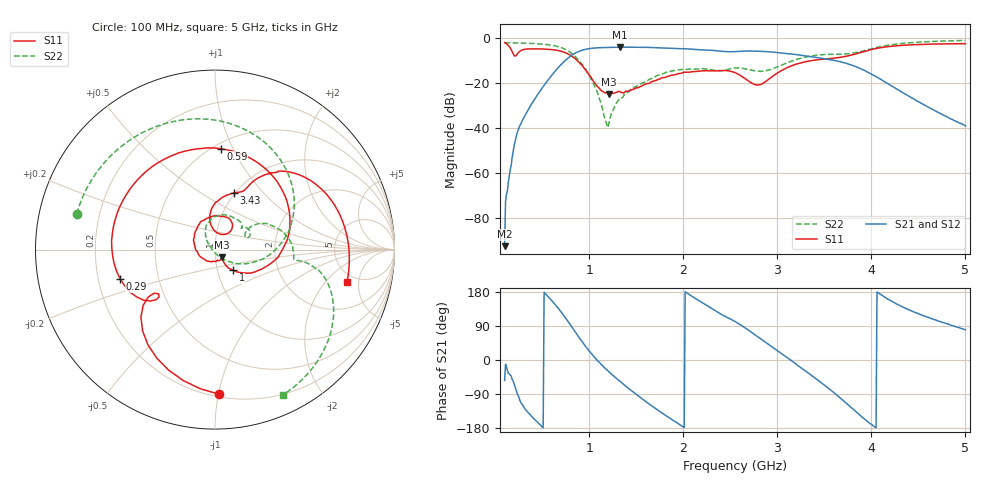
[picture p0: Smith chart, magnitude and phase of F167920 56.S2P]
!  2-Port S-parameters saved by WinCal
! VAR MeasName=S-Parameters (CALIBRATED_DATA) read from VNA (N5242A)
! VAR MeasDate=2016-11-22 9:58:16
! VAR NAME=F167920 56
! VAR FILENAME=F167920 56.S2P
! VAR DATE=2016-11-22 9:58:16
! VAR PHYS_PORTS=1,2
# Hz S DB R 50
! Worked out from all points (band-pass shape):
!   491 points, 100 MHz to 5 GHz, reference 50 ohm
!   highest |S21| = -3.95 dB at 1.33 GHz (marker M1); lowest = -92.6 dB at 100 MHz (marker M2)
!   |S21| within 3 dB of the highest: 838.6 MHz to 3.138 GHz (2.299 GHz wide, 116 % of centre)
!   lowest |S11| = -24.7 dB at 1.21 GHz (marker M3), VSWR 1.12, Z = 53.7 - j4.7 ohm
!   |S11| at or under -10 dB: 873.3 MHz to 3.356 GHz (2.483 GHz wide, 117 % of centre)
!   |S22| runs from -39.7 to -1.0 dB; largest |S21 - S12| = 0.001
!   S11 on the Smith chart (normalised r, x): 100 MHz: 0.22, -1.01; 290 MHz: 0.29, -0.14; 590 MHz: 0.54, +0.90; 1 GHz: 1.19, -0.28; 3.43 GHz: 0.99, +0.70; 5 GHz: 4.20, -3.51
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1e8  -1.86 -88.2  -92.59 -53.9  -80.56 1.6  -1.98 165.5
1.5e8  -3.76 -125.2  -61.21 -36.2  -61.52 -49.6  -2.01 158.2
2e8  -7.59 -144.4  -48.13 -62.1  -48.26 -63.1  -2.05 150.8
2.9e8  -5.14 -162.8  -36.46 -118.8  -36.55 -119.0  -2.15 137.0
4.1e8  -4.71 148.4  -27.74 -154.5  -27.73 -154.7  -2.36 117.3
5.9e8  -4.98 86.8  -17.07 160.0  -17.06 160.0  -3.05 81.9
7.5e8  -6.51 30.1  -9.71 110.3  -9.70 110.3  -5.05 40.0
9.2e8  -11.88 -29.3  -5.37 50.0  -5.36 50.0  -11.43 -11.6
1e9  -16.37 -48.9  -4.62 23.7  -4.62 23.7  -16.51 -31.9
1.18e9  -24.31 -47.7  -4.10 -24.4  -4.10 -24.4  -37.56 -120.5
1.21e9  -24.75 -48.9  -4.07 -31.5  -4.06 -31.5  -37.79 -172.5
1.33e9  -23.96 -72.6  -3.95 -57.3  -3.95 -57.3  -27.26 135.6
1.74e9  -18.24 161.5  -4.25 -134.0  -4.25 -134.0  -16.35 105.8
2.07e9  -15.10 107.9  -4.83 171.8  -4.83 171.8  -13.72 63.4
2.55e9  -15.27 55.6  -5.92 101.7  -5.93 101.6  -13.24 31.5
2.8e9  -20.75 75.7  -5.77 60.1  -5.77 60.1  -14.66 22.0
3.08e9  -13.59 97.0  -6.67 10.6  -6.68 10.6  -11.35 31.5
3.37e9  -9.89 75.3  -8.27 -41.8  -8.27 -41.8  -7.80 10.9
3.43e9  -9.55 71.4  -8.64 -52.8  -8.65 -52.8  -7.48 6.1
3.81e9  -7.23 60.7  -12.23 -130.8  -12.23 -130.8  -6.59 -7.5
4.19e9  -3.66 36.0  -20.58 158.7  -20.60 158.7  -3.03 -22.0
5e9  -2.42 -13.6  -39.06 79.8  -39.01 79.8  -0.98 -65.0
